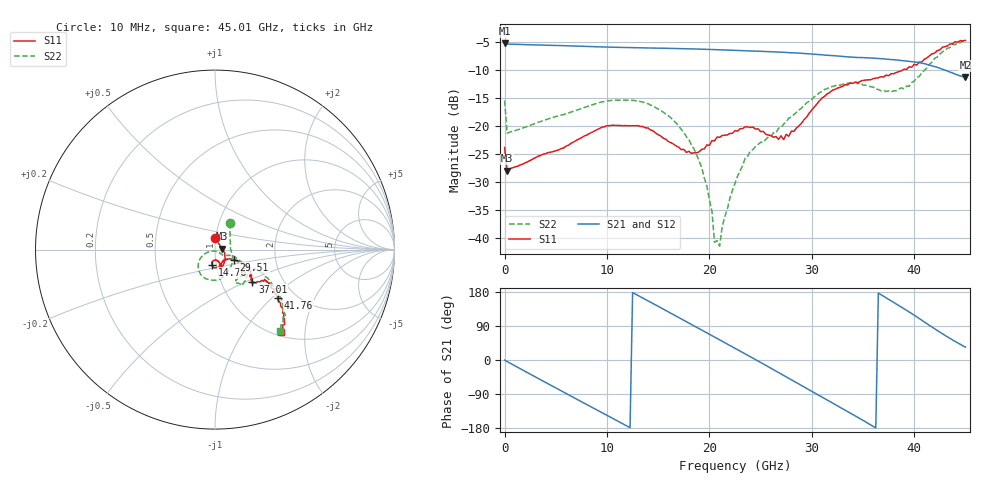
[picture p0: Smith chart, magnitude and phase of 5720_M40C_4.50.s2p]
! Device:  ADRF5720
! Description: 0.5dB LSB GaAs MMIC 6-bit Digital Attenuator
! Frequency:  0.000009 -  40 GHz
! Ports:
!	RF1	= Port 1
!	RF2	= Port 2
! Vdd:  3.3 Volt
! Vss:  -3.3 Volt
! Control:  0/3.3 Volt
! State:  4.50 dB attenuation
! Data:  The device was measured using G-S-G Probes on a matrix board.
!  Data was collected using an calibrated 4 port network analyzer.
!  The reference plane for this measurement is at the launchers.
! Note:  Analog Devices supplies this data as a sample of measured data
!  for this product.  Your particular data for this product may vary.
!  Data was taken at -40 degrees C.
!  Analog Devices reserves the right to change this data at anytime.
# GHZ S DB R 45.0
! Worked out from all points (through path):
!   181 points, 10 MHz to 45.01 GHz, reference 45 ohm
!   highest |S21| = -5.14 dB at 10 MHz (marker M1); lowest = -11.2 dB at 45.01 GHz (marker M2)
!   group delay of S21, straight-line fit = 42 ps
!   lowest |S11| = -28.0 dB at 260 MHz (marker M3), VSWR 1.08, Z = 48.7 + j0.494 ohm
!   |S11| at or under -10 dB: start of sweep to 38.83 GHz
!   |S22| runs from -41.5 to -4.7 dB; largest |S21 - S12| = 0.0021
!   S11 on the Smith chart (normalised r, x): 10 MHz: 0.99, +0.13; 14.76 GHz: 0.95, -0.16; 29.51 GHz: 1.23, -0.15; 37.01 GHz: 1.40, -0.55; 41.76 GHz: 1.63, -1.10; 45.01 GHz: 1.08, -1.49
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0.01  -23.80 89.6  -5.14 -0.5  -5.16 -0.5  -15.41 61.0
0.26  -27.97 7.3  -5.31 -4.1  -5.32 -4.1  -21.25 1.8
4.26  -24.72 -19.4  -5.52 -62.8  -5.54 -62.9  -18.68 -31.6
7.76  -21.78 -47.4  -5.71 -113.6  -5.72 -113.7  -16.67 -62.7
11.26  -19.87 -75.9  -5.90 -164.1  -5.92 -164.2  -15.36 -94.7
14.76  -21.21 -101.3  -6.03 145.3  -6.05 145.2  -16.68 -127.7
15.26  -21.76 -102.8  -6.04 137.9  -6.06 137.9  -17.19 -132.4
18.76  -24.76 -83.3  -6.19 86.5  -6.21 86.4  -25.10 -157.9
19.76  -23.35 -75.7  -6.25 71.7  -6.27 71.6  -30.66 -156.7
20.26  -22.57 -73.2  -6.28 64.3  -6.30 64.2  -35.24 -148.5
20.51  -22.62 -72.3  -6.30 60.6  -6.32 60.5  -40.76 -132.6
21.01  -22.00 -71.4  -6.33 53.1  -6.34 53.1  -41.46 -62.2
22.76  -20.88 -73.8  -6.45 27.1  -6.47 27.1  -28.95 -32.8
24.01  -20.22 -71.6  -6.54 8.6  -6.56 8.5  -24.43 -34.0
27.26  -22.39 -49.2  -6.79 -40.4  -6.81 -40.6  -19.63 -19.1
29.51  -18.36 -28.8  -7.02 -74.9  -7.04 -75.1  -15.83 -25.0
30.26  -16.56 -26.0  -7.12 -86.5  -7.14 -86.6  -14.71 -28.9
34.01  -12.34 -36.5  -7.65 -143.8  -7.68 -144.0  -12.30 -48.9
37.01  -11.19 -40.9  -7.95 168.4  -7.97 168.2  -13.58 -55.5
37.76  -10.60 -39.3  -8.08 156.1  -8.10 155.9  -13.89 -51.2
41.76  -7.06 -37.5  -9.19 86.8  -9.21 86.6  -8.53 -31.3
45.01  -4.66 -51.4  -11.25 33.9  -11.28 33.8  -4.71 -51.1
